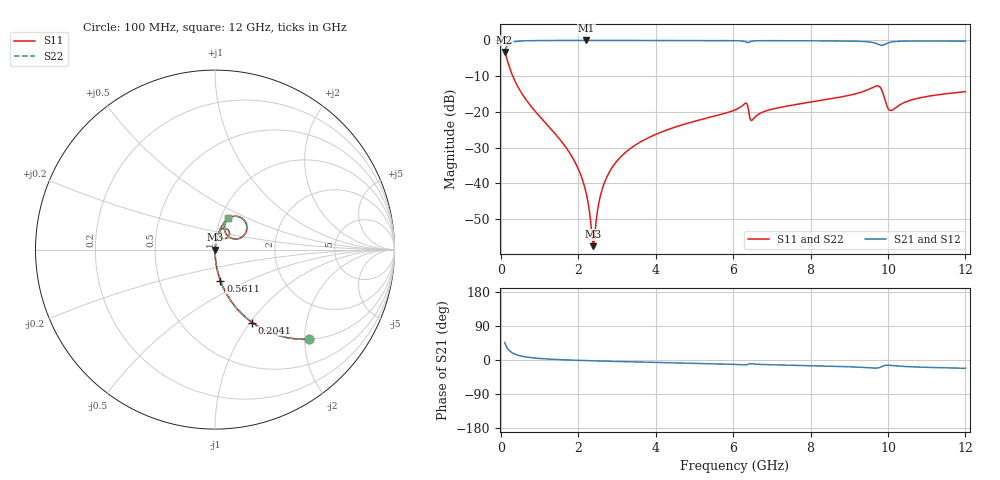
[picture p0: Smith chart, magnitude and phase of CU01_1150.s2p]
! S-parameter model data by Modelithics Inc. support@modelithics.com 813-866-6335 Tampa FL USA
! S-Parameter data specifications:
! Substrate: 20-mil Rogers, substrate thickness, H=0.508mm, Dielectric constant, Er=3.75
! PCB Mounting Pad Footprint: Pad width, PadW=0.35mm , Pad length, PadL=0.30mm , Pad gap, PadG (edge-to-edge)=0.25mm , Reference planes=0.85mm apart
! Created Tue May  8 14:01:25 2018
# hz S ma R 50
! 2 Port Network Data from SP1.SP block
! freq  magS11  angS11  magS21  angS21  magS12  angS12  magS22  angS22
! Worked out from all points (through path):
!   801 points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, 100 MHz to 12 GHz, reference 50 ohm
!   highest |S21| = -0.01 dB at 2.212 GHz (marker M1); lowest = -3.3 dB at 100 MHz (marker M2)
!   group delay of S21, straight-line fit = 7.1 ps
!   lowest |S11| = -57.6 dB at 2.391 GHz (marker M3), VSWR 1.00, Z = 50.1 - j0.00875 ohm
!   |S11| at or under -10 dB: 311.5 MHz to end of sweep
!   |S22| runs from -57.6 to -2.8 dB; largest |S21 - S12| = 0
!   S11 on the Smith chart (normalised r, x): 100 MHz: 1.00, -2.11; 204.1 MHz: 1.00, -1.03; 561.1 MHz: 1.00, -0.36; 12 GHz: 1.09, +0.40
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1e8  0.7255 -43.5  0.6878 46.4  0.6878 46.4  0.7255 -43.5
2.04125e8  0.4569 -62.9  0.889 27.0  0.889 27.0  0.4569 -62.9
3.38e8  0.2928 -73.2  0.9556 16.7  0.9556 16.7  0.2928 -73.2
5.61125e8  0.1751 -80.2  0.9838 9.6  0.9838 9.6  0.1751 -80.2
1.691625e9  0.03127 -87.7  0.9984 0.3  0.9984 0.3  0.03127 -87.7
2.09325e9  0.01191 -85.3  0.9987 -1.2  0.9987 -1.2  0.01191 -85.3
2.21225e9  0.007039 -81.2  0.9987 -1.6  0.9987 -1.6  0.007039 -81.2
2.346125e9  0.002148 -54.8  0.9987 -2.0  0.9987 -2.0  0.002148 -54.8
2.39075e9  0.001312 -3.8  0.9987 -2.2  0.9987 -2.2  0.001312 -3.8
2.599e9  0.007513 76.8  0.9986 -2.8  0.9986 -2.8  0.007513 76.8
2.86675e9  0.01626 81.4  0.9984 -3.5  0.9984 -3.5  0.01626 81.4
3.34275e9  0.03046 82.3  0.9979 -4.8  0.9979 -4.8  0.03046 82.3
4.071625e9  0.05006 81.5  0.997 -6.6  0.997 -6.6  0.05006 81.5
6.05e9  0.1062 76.0  0.9898 -11.6  0.9898 -11.6  0.1062 76.0
6.31775e9  0.1318 62.9  0.9598 -13.1  0.9598 -13.1  0.1318 62.9
6.49625e9  0.07672 65.0  0.9774 -10.1  0.9774 -10.1  0.07672 65.0
6.91275e9  0.1054 75.9  0.991 -12.3  0.991 -12.3  0.1054 75.9
8.04325e9  0.1379 73.5  0.9872 -15.2  0.9872 -15.2  0.1379 73.5
9.724125e9  0.2306 47.6  0.893 -21.2  0.893 -21.2  0.2306 47.6
9.82825e9  0.2087 32.2  0.8535 -18.1  0.8535 -18.1  0.2087 32.2
1.002162e10  0.1077 37.9  0.9298 -13.9  0.9298 -13.9  0.1077 37.9
1.2e10  0.1914 67.0  0.9777 -21.9  0.9777 -21.9  0.1914 67.0
